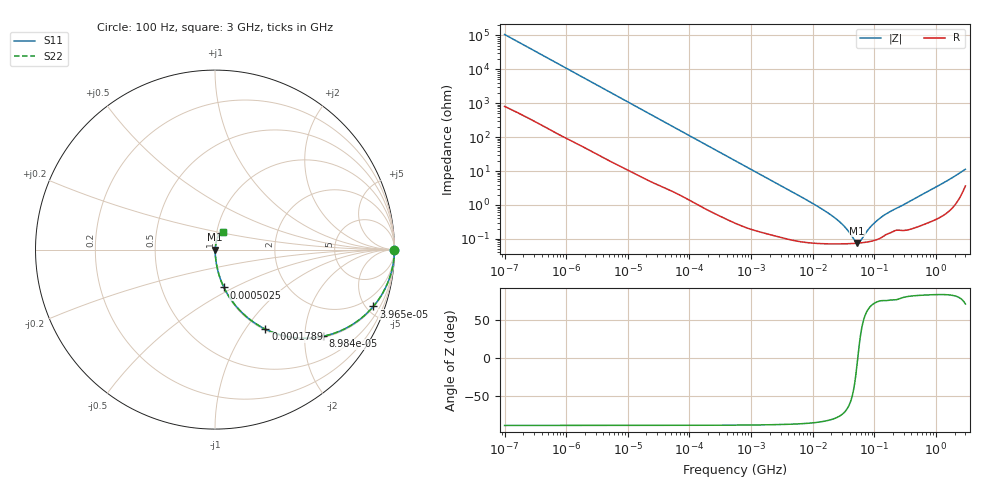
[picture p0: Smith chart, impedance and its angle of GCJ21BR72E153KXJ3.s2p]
!Murata Part Number: GCJ21BR72E153KXJ3
!These Parameters are Measured in Series Mode Connection
!Data Generated on Mar 13, 2026
!  o--ll--o
!Port1  Port2
!  o------o
!Operation Temp=25[degC], DC Bias Voltage=0[V]
!Freq. Start=100[Hz] Stop=3[GHz] 401[Steps]
# Hz S RI R 50
!Freq.(Hz) S11(Real) S11(Imag) S21(Real) S21(Imag) S12(Real) S12(Imag) S22(Real) S22(Imag)
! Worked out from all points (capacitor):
!   401 points, 100 Hz to 3 GHz, reference 50 ohm
!   read as one part in series: C = 15 nF near 109 Hz
!   lowest |Z| = 75.3 mohm at 52.48 MHz (marker M1)
!   series resonance near 53.82 MHz, so ESL is about 580 pH
!   S11 on the Smith chart (normalised r, x): 100 Hz: open; 39.66 kHz: 1.06, -5.54; 89.84 kHz: 1.03, -2.46; 178.9 kHz: 1.02, -1.24; 502.5 kHz: 1.01, -0.45; 3 GHz: 1.07, +0.21
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100  1 -0.000942  8e-06 0.000942  8e-06 0.000942  1 -0.000942
1788  0.9996 -0.0166  0.000423 0.0166  0.000423 0.0166  0.9996 -0.0166
9582  0.9915 -0.0872  0.00852 0.0872  0.00852 0.0872  0.9915 -0.0872
31977  0.9192 -0.2671  0.0808 0.2671  0.0808 0.2671  0.9192 -0.2671
39655  0.8819 -0.317  0.1181 0.317  0.1181 0.317  0.8819 -0.317
58416  0.7779 -0.4096  0.2221 0.4096  0.2221 0.4096  0.7779 -0.4096
89839  0.6014 -0.4834  0.3986 0.4834  0.3986 0.4834  0.6014 -0.4834
178874  0.2812 -0.4434  0.7188 0.4434  0.7188 0.4434  0.2812 -0.4434
287190  0.1343 -0.3346  0.8657 0.3346  0.8657 0.3346  0.1343 -0.3346
502545  0.05 -0.2111  0.95 0.2111  0.95 0.2111  0.05 -0.2111
547723  0.0427 -0.1953  0.9573 0.1953  0.9573 0.1953  0.0427 -0.1953
1750920  0.00555 -0.064  0.9945 0.064  0.9945 0.064  0.00555 -0.064
9794414  0.000878 -0.0113  0.9991 0.0113  0.9991 0.0113  0.000878 -0.0113
2.635803e7  0.000721 -0.0033  0.9993 0.0033  0.9993 0.0033  0.000721 -0.0033
3.412477e7  0.00072 -0.002  0.9993 0.002  0.9993 0.002  0.00072 -0.002
4.815176e7  0.000736 -0.000473  0.9993 0.000473  0.9993 0.000473  0.000736 -0.000473
5.248048e7  0.000745 -0.000106  0.9993 0.000106  0.9993 0.000106  0.000745 -0.000106
5.9714e7  0.000761 0.000443  0.9992 -0.000443  0.9992 -0.000443  0.000761 0.000443
7.730952e7  0.000812 0.00157  0.9992 -0.00157  0.9992 -0.00157  0.000812 0.00157
1.000898e8  0.000906 0.00281  0.9991 -0.00281  0.9991 -0.00281  0.000906 0.00281
1.751444e8  0.0015 0.00597  0.9985 -0.00597  0.9985 -0.00597  0.0015 0.00597
3e9  0.0452 0.0984  0.9548 -0.0984  0.9548 -0.0984  0.0452 0.0984
